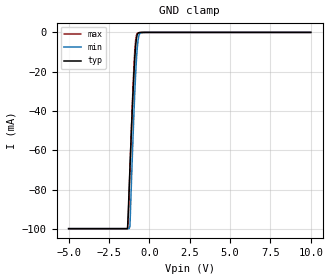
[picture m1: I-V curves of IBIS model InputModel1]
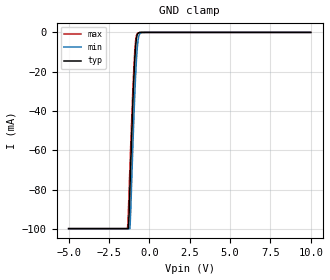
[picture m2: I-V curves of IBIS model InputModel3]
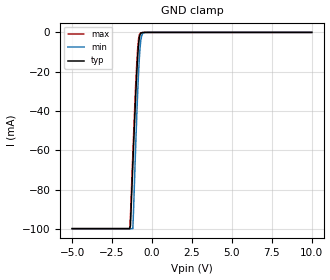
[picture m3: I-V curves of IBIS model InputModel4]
[IBIS Ver]   2.1
[File name]   e_016xd5.ibs   | e_= TSOP, f016xd= abbr chip name, 5= 5V Vcc
[File Rev]   2.40
[Date]   13-February-96
[Source]   File generated from lab measurements at Intel Corporation
[Notes]   Rev 2.00 fixes simulation model flaw.
   Rev 2.01 fixes typo errors in comments only.
   Rev 2.10 adds two omitted comment markers (|) to InputModel1
   and implements improvements for Quad parser IBIS2XTK:
   * adds zero current [POWER_clamp] to input models
   * changes model name from "I/O" to "InputOutput"
   * changes model type "Open_Drain" to "Open_drain"
   Rev 2.20 adds required dV/dt_r for OpenDrainOutput.
   Rev 2.30 adds 3/5# pin to pin #1.  The input model remains the
   same as it was included in rev 2.20, though the pin
   was a no connect in that model.
   Rev 2.40 All data was replaced by actual measurements
   performed in a lab.
[Disclaimer] INTEL DEVELOPER'S SOFTWARE LICENSE AGREEMENT
| BY USING THIS SOFTWARE, YOU ARE AGREEING TO BE BOUND
| BY THE TERMS OFTHIS AGREEMENT.  DO NOT USE THE SOFTWARE
| UNTIL YOU HAVE CAREFULLY READAND AGREED TO THE FOLLOWING
| TERMS AND CONDITIONS.  IF YOU DO NOT AGREETO THE TERMS
| OF THIS AGREEMENT, PROMPTLY RETURN THE SOFTWARE PACKAGE
| ANDANY ACCOMPANYING ITEMS.
| IF YOU USE THIS SOFTWARE, YOU WILL BE BOUND BY THE TERMS
| OF THIS AGREEMENT
| LICENSE: Intel Corporation ("Intel") grants you the non-exclusive right
| to use the enclosed software program ("Software").  You will not use,
| copy, modify, rent, sell or transfer the Software or any portion
| thereof, except as provided in this Agreement.
| System OEM Developers may:
| 1.   Copy the Software for support, backup or archival purposes;
| 2.   Install, use, or distribute Intel owned Software in object code
|   only;
| 3.   Modify and/or use Software source code that Intel directly makes
|   available to you as an OEM Developer;
| 4.   Install, use, modify, distribute, and/or make or have made
|   derivatives ("Derivatives") of Intel owned Software under the
|   terms and conditions in this Agreement, ONLY if you are a System
|   OEM Developer and NOT an end-user.
| RESTRICTIONS:
| YOU WILL NOT:
| 1.   Copy the Software, in whole or in part, except as provided for
|   in this Agreement;
| 2.   Decompile or reverse engineer any Software provided in object
|   code format;
| 3.   Distribute any Software or Derivative code to any end-users,
|   unless approved by Intel in a prior writing.
| TRANSFER: You may transfer the Software to another OEM
| Developer if thereceiving party agrees to the terms of this
| Agreement at the sole risk of any receiving party.
| OWNERSHIP AND COPYRIGHT OF SOFTWARE:
| Title to the Software and all copies thereof remain with Intel
| or its vendors.  The Software iscopyrighted and is protected by
| United States and international copyright laws.  You will not
| remove the copyright notice from the Software.  You agree to
| prevent any unauthorized copying of the Software.
| DERIVATIVE WORK: OEM Developers that make or have made
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[Copyright]   Copyright 1995,1996, Intel Corporation, All Rights Reserved
[Component]   E28F016XD   | 56-lead TSOP package, 28F016XD
[Manufacturer]  Intel   | DRAM-Interface Flash Memory
|   | operating in 5V Vcc range
[Package]
|The following values apply for the Copper leadframe.
|Variable   typ   min   max
  R_pkg   48m   41m   54m
  L_pkg   4.92nH   4.44nH   5.39nH
  C_pkg   0.48pF   0.45pF   0.50pF
|The following values apply for the Alloy-42 leadframe.
| R_pkg   195m   180m   210m
| L_pkg   4.92nH   4.44nH   5.39nH
| C_pkg   0.48pF   0.45pF   0.50pF
|**********************Pin Defintion***********************************
[Pin]  signal_name   model_name   R_pin   L_pin   C_pin
  1   3/5#   InputModel1
  2   GND   InputModel1
  3   NC   InputModel2
  4   A9   InputModel3
  5   A8   InputModel3
  6   A7   InputModel1
  7   A6   InputModel1
  8   A5   InputModel1
  9   VCC   POWER
 10   RAS#   InputModel1
 11   CAS#   InputModel3
 12   NC   InputModel1
 13   NC   InputModel1
 14   GND   InputModel1
 15   VPP   POWER
 16   RP#   InputModel4
 17   NC   InputModel1
 18   NC   InputModel1
 19   NC   InputModel1
 20   NC   InputModel1
 21   GND   GND
 22   NC   InputModel1
 23   NC   InputModel1
 24   A4   InputModel1
 25   A3   InputModel1
 26   A2   InputModel1
 27   A1   InputModel1
 28   A0   InputModel1
 29   NC   InputModel5
 30   NC   InputModel5
 31   VCC   InputModel1
 32   NC   InputModel1
 33   DQ0   InputOutput
 34   DQ8   InputOutput
 35   DQ1   InputOutput
 36   DQ9   InputOutput
 37   VCC   POWER
 38   DQ2   InputOutput
 39   DQ10   InputOutput
 40   DQ3   InputOutput
 41   DQ11   InputOutput
 42   GND   GND
 43   VCC   POWER
 44   DQ4   InputOutput
 45   DQ12   InputOutput
 46   DQ5   InputOutput
 47   DQ13   InputOutput
 48   GND   GND
 49   DQ6   InputOutput
 50   DQ14   InputOutput
 51   DQ7   InputOutput
 52   DQ15   InputOutput
 53   RY/BY#   OpenDrainOutput
 54   OE#   InputModel1
 55   WE#   InputModel4
 56   WP#   InputModel1
|*********************Input Model 2***************************************
[Model]   InputModel2
Model_type   Input
|   Model for pin3(NC)
Vinl = 0.8V
Vinh = 2.0V
|Variable   typ   min   max
C_comp   5.61p   NA   7.6p
[Voltage Range]   5.0V   4.5V   5.5V
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| Models and submodels in the file (7): InputModel1 (Input), InputModel2 (Input), InputModel3 (Input), InputModel4 (Input), InputModel5 (Input), InputOutput (I/O), OpenDrainOutput (Open_drain)
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|***********************Input Model 1*********************************
[Model]   InputModel1
Model_type   Input
|   Model for pin1(3/5#), pin2(GND), pin12(NC), pin13(NC),
|   pin14(GND), pin17(NC), pin18(NC), pin19(NC), pin20(NC),
|   pin22(NC), pin23(NC), pin31(VCC), pin32(NC), OE#,
|   WP#, A[7:0], and RAS#.
Vinl = 0.8V
Vinh = 2.0V
|Variable   typ   min   max
C_comp   5.61p   NA   7.6p
[Voltage Range]   5.0V   4.5V   5.5V
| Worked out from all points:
|   GND clamp passes 1 mA (typ) near -0.74 V on its own axis
[GND_clamp]
|Voltage   I(typ)   I(min)   I(max)
-5V       -99.85mA   -99.85mA   -99.85mA
-1.35V    -99.85mA   -99.85mA   -99.85mA
-1.3V     -90.3mA    -99.85mA   -94.33mA
-1.2V     -68.5mA    -98.37mA   -69.77mA
-1.05V    -37.91mA   -62.21mA   -35.67mA
-950mV    -20.05mA   -40.17mA   -16.43mA
-900mV    -12.63mA   -30.22mA   -9.019mA
-850mV    -6.881mA   -21.47mA   -4.01mA
-750mV    -1.101mA   -7.938mA   -497.3uA
-650mV    -190.2uA   -1.778mA   -141.6uA
-500mV    -22.36uA   -107.9uA   -13.27uA
10V       0A         0A         0A
[POWER_clamp]
| Input buffer circuits of this product do not intrinsically
| require a [POWER_clamp] definition.  This zero current
| [POWER_clamp] is provided for compatibility with some ibis
| parsers.
|Voltage  I(typ)   I(min)   I(max)
-5V       0A         0A         0A
0V        0A         0A         0A
5V        0A         0A         0A
10V       0A         0A         0A
|*******************Input Model 3*********************************
[Model]   InputModel3
Model_type   Input
|   for A[9], A[8], CAS#
Vinl = 0.8V
Vinh = 2.0V
|Variable   typ   min   max
C_comp   5.61p   NA   7.6p
[Voltage Range]   5.0V   4.5V   5.5V
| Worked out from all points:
|   GND clamp passes 1 mA (typ) near -0.74 V on its own axis
[GND_clamp]
|Voltage I(typ)   I(min)   I(max)
-5V       -99.83mA   -99.86mA   -99.85mA
-1.35V    -99.83mA   -99.86mA   -99.85mA
-1.3V     -99.83mA   -99.86mA   -91.19mA
-1.25V    -91.84mA   -99.86mA   -79.26mA
-1.2V     -79.02mA   -99.86mA   -67.68mA
-1V       -31.01mA   -53.1mA    -25.08mA
-950mV    -22.07mA   -41.74mA   -16.28mA
-850mV    -7.219mA   -22.07mA   -4.133mA
-750mV    -1.138mA   -8.043mA   -576uA
-650mV    -229.5uA   -1.811mA   -181.7uA
-500mV    0A         -129.1uA   -19.82uA
10V       0A         0A         0A
[POWER_clamp]
| Input buffer circuits of this product do not intrinsically
| require a [POWER_clamp] definition.  This zero current
| [POWER_clamp] is provided for compatibility with some ibis
| parsers.
|Voltage  I(typ)   I(min)   I(max)
-5V       0A         0A         0A
0V        0A         0A         0A
5V        0A         0A         0A
10V       0A         0A         0A
|******************Input Model 4*********************************
[Model]   InputModel4
Model_type   Input
|   Model for RP#, WE#
Vinl = 0.8V
Vinh = 2.0V
|Variable   typ   min   max
C_comp   5.61p   NA   7.6p
[Voltage Range]   5.0V   4.5V   5.5V
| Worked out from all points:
|   GND clamp passes 1 mA (typ) near -0.74 V on its own axis
[GND_clamp]
|Voltage I(typ)   I(min)   I(max)
-5V       -99.84mA   -99.85mA   -99.84mA
-1.4V     -99.84mA   -99.85mA   -99.84mA
-1.35V    -98.45mA   -99.85mA   -93.48mA
-1.2V     -67.39mA   -99.85mA   -61.9mA
-1.15V    -57.12mA   -89.14mA   -51.65mA
-1.05V    -37.56mA   -64.46mA   -31.14mA
-950mV    -19.93mA   -41.4mA    -15.11mA
-850mV    -6.868mA   -21.92mA   -3.833mA
-750mV    -1.126mA   -7.98mA    -496.7uA
-650mV    -193.8uA   -1.793mA   -141.7uA
-500mV    -22.97uA   -113.7uA   -13.69uA
10V       0A         0A         0A
[POWER_clamp]
| Input buffer circuits of this product do not intrinsically
| require a [POWER_clamp] definition.  This zero current
| [POWER_clamp] is provided for compatibility with some ibis
| parsers.
|Voltage  I(typ)   I(min)   I(max)
-5V       0A         0A         0A
0V        0A         0A         0A
5V        0A         0A         0A
10V       0A         0A         0A
